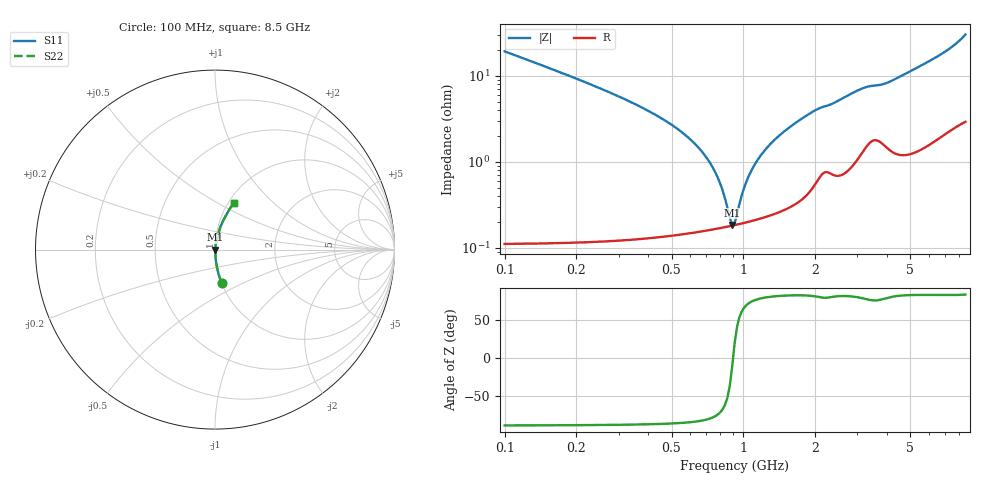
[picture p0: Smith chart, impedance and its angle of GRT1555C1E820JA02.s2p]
!Murata Part Number: GRT1555C1E820JA02
!These Parameters are Measured in Series Mode Connection
!Data Generated on Jun 19, 2026
!  o--ll--o
!Port1  Port2
!  o------o
!Operation Temp=25[degC], DC Bias Voltage=0[V]
!Freq. Start=100[MHz] Stop=9[GHz] 401[Steps]
# Hz S RI R 50
!Freq.(Hz) S11(Real) S11(Imag) S21(Real) S21(Imag) S12(Real) S12(Imag) S22(Real) S22(Imag)
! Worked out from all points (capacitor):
!   401 points, 100 MHz to 8.5 GHz, reference 50 ohm
!   read as one part in series: C = 82 pF near 142 MHz
!   lowest |Z| = 185 mohm at 898 MHz (marker M1)
!   series resonance near 904.8 MHz, so ESL is about 380 pH
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1e8  0.0364 -0.1845  0.9636 0.1845  0.9636 0.1845  0.0364 -0.1845
2.68e8  0.00552 -0.0656  0.9945 0.0656  0.9945 0.0656  0.00552 -0.0656
5.83e8  0.00184 -0.0194  0.9982 0.0194  0.9982 0.0194  0.00184 -0.0194
6.88e8  0.00171 -0.0118  0.9983 0.0118  0.9983 0.0118  0.00171 -0.0118
7.72e8  0.00171 -0.00681  0.9983 0.00681  0.9983 0.00681  0.00171 -0.00681
8.56e8  0.00177 -0.00237  0.9982 0.00237  0.9982 0.00237  0.00177 -0.00237
8.77e8  0.00179 -0.00133  0.9982 0.00133  0.9982 0.00133  0.00179 -0.00133
8.98e8  0.00181 -0.000322  0.9982 0.000322  0.9982 0.000322  0.00181 -0.000322
9.19e8  0.00184 0.000666  0.9982 -0.000666  0.9982 -0.000666  0.00184 0.000666
9.4e8  0.00187 0.00163  0.9981 -0.00163  0.9981 -0.00163  0.00187 0.00163
1.024e9  0.002 0.00531  0.998 -0.00531  0.998 -0.00531  0.002 0.00531
1.066e9  0.00208 0.00706  0.9979 -0.00706  0.9979 -0.00706  0.00208 0.00706
1.129e9  0.00221 0.00957  0.9978 -0.00957  0.9978 -0.00957  0.00221 0.00957
1.297e9  0.00263 0.0158  0.9974 -0.0158  0.9974 -0.0158  0.00263 0.0158
1.507e9  0.00334 0.0231  0.9967 -0.0231  0.9967 -0.0231  0.00334 0.0231
2.011e9  0.00715 0.0391  0.9928 -0.0391  0.9928 -0.0391  0.00715 0.0391
2.914e9  0.0133 0.0624  0.9867 -0.0624  0.9867 -0.0624  0.0133 0.0624
3.25e9  0.0193 0.0696  0.9807 -0.0696  0.9807 -0.0696  0.0193 0.0696
4.3e9  0.0201 0.087  0.9799 -0.087  0.9799 -0.087  0.0201 0.087
5.707e9  0.0317 0.1299  0.9683 -0.1299  0.9683 -0.1299  0.0317 0.1299
7.114e9  0.0557 0.1806  0.9443 -0.1806  0.9443 -0.1806  0.0557 0.1806
8.5e9  0.1042 0.2608  0.8958 -0.2608  0.8958 -0.2608  0.1042 0.2608
